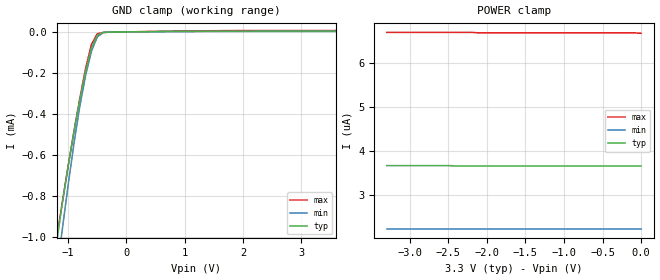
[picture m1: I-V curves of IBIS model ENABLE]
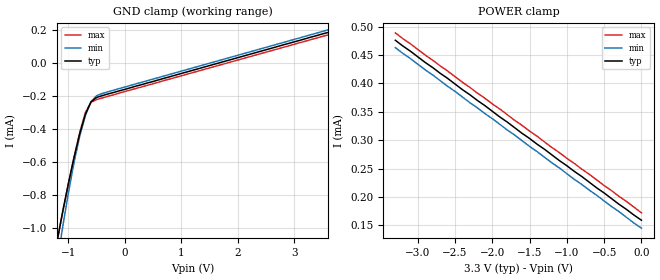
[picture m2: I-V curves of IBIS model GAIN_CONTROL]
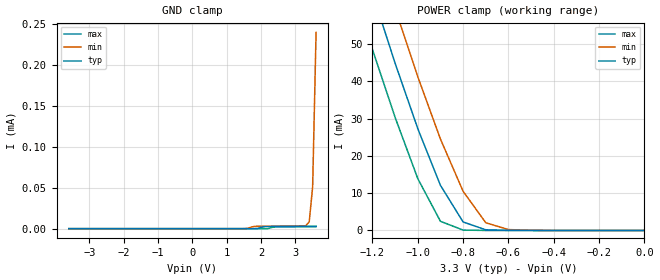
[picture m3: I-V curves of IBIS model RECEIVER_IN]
|   Texas Instruments Incorporated
|   Data Transmissions Products
|   IBIS Model for SN65LVDS19
|   8DRF  Small-Outline No-Lead Package
[IBIS Ver]   3.2
[Comment char]   |_char
[File name]   lvds17_gc_vcc.ibs
[File Rev]   1.1
[Date]   9Sep04
[Source]   File originated at Texas Instruments Incorporated.
   Data Transmission Products Group.
[Notes]
[Disclaimer]
(C) Copyright Texas Instruments Incorporated 2004
   All rights reserved
  Texas Instruments Incorporated hereby grants the user of this IBIS
model a non-exclusive, nontransferable license to use this IBIS model
under the following terms.  Before using this IBIS model, the user
should read this license.  If the user does not accept these terms,
the IBIS model should be returned to Texas Instruments within 30 days.
  The user is granted this license only to use the IBIS model and
is not granted rights to sell, load, rent, lease or license the IBIS
model in whole or in part, or in modified form to anyone other than
user.  User may modify the IBIS model to suit its specific applications
but rights to derivative works and such modifications shall belong to
Texas Instruments.
  This IBIS model is provided on an "AS IS" basis and Texas Instruments
makes absolutely no warranty with respect to the information contained
herein.  TEXAS INSTRUMENTS DISCLAIMS AND CUSTOMER WAIVES ALL WARRANTIES,
EXPRESS OR IMPLIED, INCLUDING WARRANTIES OF MERCHANTABILITY OR FITNESS
FOR A PARTICULAR PURPOSE. The entire risk as to quality and performance
is with the Customer. ACCORDINGLY, IN NO EVENT SHALL THE COMPANY BE LIABLE
FOR ANY DAMAGES, WHETHER IN CONTRACT OR TORT,INCLUDING ANY LOST PROFITS
OR OTHER INCIDENTAL, CONSEQUENTIAL, EXEMPLARY, OR PUNITIVE DAMAGES ARISING
OUT OF THE USE OR APPLICATION OF THE IBIS model provided in this package.
Further, Texas Instruments reserves the right to discontinue or make changes
without notice to any product herein to improve reliability, function, or
design. Texas Instruments does not convey any license under patent rights
or any other intellectual property rights, including those of third parties.
Contact Texas Instruments at ATTN:DATA TRANSMISSIONS
[Copyright]   Copyright 2004, Texas Instruments, All Rights Reserved
[Component]   LVDS17DRF
[Manufacturer]  Texas Instruments Incorporated
[Package]
|   typ   min   max
R_pkg   0.189   0.176   0.203
L_pkg   0.802nH   0.759nH   0.850nH
C_pkg   0.053pF   0.046pF   0.067pF
[Pin]   signal_name   model_name   R_pin   L_pin   C_pin
1   Q/   LOW_GAIN_QBAR_VCC  0.194   0.817n   0.054p
2   A   RECEIVER_IN   0.193   0.814n   0.054p
3   B   RECEIVER_IN   0.187   0.793n   0.052p
4   GC   GAIN_CONTROL   0.194   0.821n   0.054p
5   EN/   ENABLE   0.176   0.759n   0.046p
6   Z   HIGH_GAIN_OUT   0.188   0.799n   0.051p
7   Y   HIGH_GAIN_OUT   0.181   0.772n   0.050p
8   VCC   POWER   0.187   0.791n   0.052p
9   GND   GND   0.203   0.850n   0.067p
[Diff_pin]   inv_pin   vdiff   tdelay_typ   tdelay_min   tdelay_max
| The 'A/Y' pin is Diff_pin and the 'B/Z' pin is the inv_pin
7   6   0.000   0 0 0
2   3   0.100   0 0 0
| Models and submodels in the file (5): ENABLE (Input), GAIN_CONTROL (Input), RECEIVER_IN (Input), LOW_GAIN_QBAR_VCC (Output_ECL), HIGH_GAIN_OUT (3-state)
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|   Enable Input Model
[Model]   ENABLE
Model_type   Input
|Signals   EN/
Vinh = 2.0
Vinl = 0.8
C_comp   3.3pF   3.28pF   3.38pF
|   typ   min   max
[Temperature Range]   25   -40   85
[Voltage range]   3.3V   3.0V   3.6V
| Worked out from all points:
|   GND clamp passes 1 mA (typ) near -1.18 V on its own axis
[GND_clamp]
|Voltage I(typ)   I(min)   I(max)
-3.6V     -6.81mA    -7.03mA    -6.59mA
-1.2V     -1.03mA    -1.18mA    -1.01mA
-1.1V     -834uA     -961uA     -829uA
-1V       -652uA     -745uA     -654uA
-900mV    -485uA     -543uA     -484uA
-800mV    -330uA     -362uA     -323uA
-700mV    -191uA     -211uA     -176uA
-600mV    -78.2uA    -93.9uA    -60.7uA
-500mV    -15.7uA    -24.3uA    -8.94uA
-400mV    -2.37uA    -3.64uA    -2.58uA
-300mV    -1.1uA     -901nA     -1.79uA
3.6V      3.66uA     2.24uA     6.67uA
[Power_clamp]
| Note that the[POWER_clamp]voltage table is referenced to Vcc
| and is calculated using Vtable=Vcc - Vmeasured.
|Voltage I(typ)   I(min)   I(max)
-3.3V     3.67uA     2.24uA     6.69uA
-2.5V     3.67uA     2.24uA     6.69uA
-2.4V     3.66uA     2.24uA     6.69uA
-2.2V     3.66uA     2.24uA     6.69uA
-2.1V     3.66uA     2.24uA     6.68uA
-100mV    3.66uA     2.24uA     6.68uA
0V        3.66uA     2.24uA     6.67uA
|   Gain Control Input Model
[Model]   GAIN_CONTROL
Model_type   Input
|Signals   GC
Vinh = 2.0
Vinl = 0.8
C_comp   3.3pF   3.28pF   3.38pF
|   typ   min   max
[Temperature Range]   25   -40   85
[Voltage range]   3.3V   3.0V   3.6V
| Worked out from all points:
|   GND clamp passes 1 mA (typ) near -1.16 V on its own axis
[GND_clamp]
|Voltage I(typ)   I(min)   I(max)
-3.6V     -6.81mA    -7.03mA    -6.59mA
-1.2V     -1.08mA    -1.21mA    -1.08mA
-1.1V     -897uA     -990uA     -903uA
-1V       -729uA     -786uA     -732uA
-900mV    -572uA     -601uA     -569uA
-800mV    -429uA     -443uA     -420uA
-700mV    -310uA     -318uA     -300uA
-600mV    -235uA     -234uA     -237uA
-500mV    -208uA     -197uA     -221uA
-100mV    -168uA     -154uA     -182uA
3.6V      187uA      203uA      172uA
[Power_clamp]
| Note that the[POWER_clamp]voltage table is referenced to Vcc
| and is calculated using Vtable=Vcc - Vmeasured.
|Voltage I(typ)   I(min)   I(max)
-3.3V     476uA      463uA      489uA
-800mV    236uA      222uA      249uA
-300mV    187uA      174uA      201uA
0V        159uA      145uA      172uA
|   Receiver Input Model
[Model]   RECEIVER_IN
Model_type   Input
|Signals   A
Vinh = 2.2
Vinl = 1.8
|   typ   min   max
C_comp   1.0pF   0.98pF   1.10pF
|   typ   min   max
[Temperature Range]   25   -40   85
[Voltage range]   3.3V   3.0V   3.6V
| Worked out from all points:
|   POWER clamp passes 1 mA (typ) near -0.74 V on its own axis
[GND_clamp]
|Voltage I(typ)   I(min)   I(max)
-3.6V     -93.5pA    -92.3pA    -96.3pA
1.5V      -4.04pA    13.2nA     -8.24pA
1.8V      4.55nA     2.8uA      -3.22pA
2.1V      2.52uA     3.01uA     483pA
2.4V      2.64uA     3.1uA      2.1uA
3.3V      2.9uA      3.61uA     2.32uA
3.4V      2.93uA     8.35uA     2.35uA
3.5V      2.96uA     51uA       2.37uA
3.6V      2.99uA     240uA      2.4uA
[Power_clamp]
| Note that the[POWER_clamp]voltage table is referenced to Vcc
| and is calculated using Vtable=Vcc - Vmeasured.
|Voltage   I(typ)   I(min)   I(max)
-3.3V     557mA      575mA      539mA
-1.3V     83.2mA     98.5mA     67.8mA
-1.2V     63.6mA     78.6mA     48.5mA
-1.1V     44.8mA     59.4mA     30.3mA
-1V       27.3mA     41.2mA     13.9mA
-900mV    12.1mA     24.5mA     2.46mA
-800mV    2.28mA     10.5mA     111uA
-700mV    181uA      2.08mA     10.4uA
-600mV    29.5uA     240uA      2.64uA
0V        2.9uA      3.29uA     2.4uA
